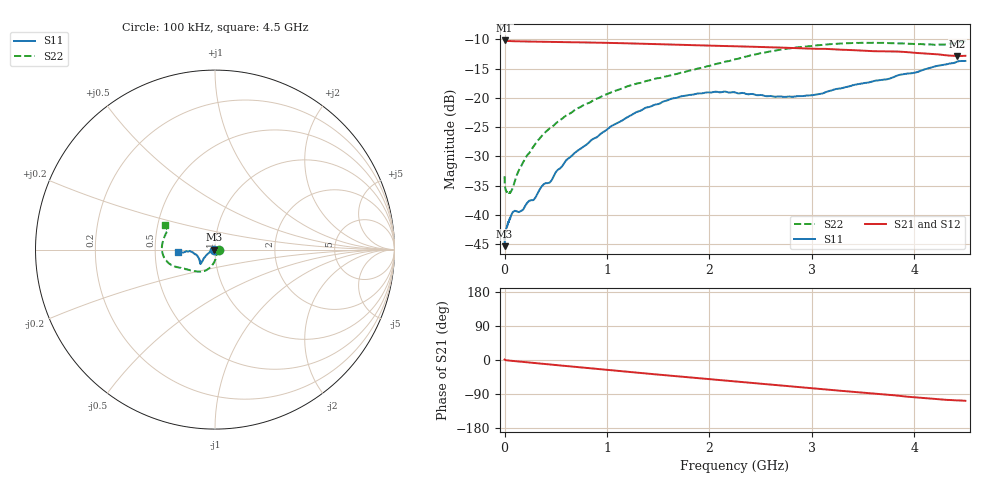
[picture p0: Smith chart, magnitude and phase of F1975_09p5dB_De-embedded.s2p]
! Integrated Device Technology
! Corporate Headquarters
! 6024 Silver Creek Valley Road
! San Jose, CA 95138  USA
! Phone:  1-408-284-8200
! Toll Free:  1-800-223-1366
! Webpage:  http://www.idt.com/
! Timing and RF Division
! 515 Groton Road, Suite 102
! Westford, MA 01886-6024
! Device:  F1975
! Description: 6-bit, 75 ohm, 0.5 dB Digital Step Attenuator
! Frequency:  5.0 MHz -  3.00 GHz
! Package:  4x4 mm QFN Plastic Package: 20 pin
! Ports:  2 RF, 11 DC
!  Pin  1  = D5 (16 dB)
!  Pin  2  = RF1  =  Port 1
!  Pin  3  = Serial Data In (DATA)
!  Pin  4  = Serial Clock (CLK)
!  Pin  5  = Serial Latch Enable (LE)
!  Pin  6  = VDD
!  Pin  7  = NC
!  Pin  8  = NC
!  Pin  9  = NC
!  Pin 10  = GND
!  Pin 11  = GND
!  Pin 12  = NC
!  Pin 13  = VMODE
!  Pin 14  = RF2  =  Port 2
!  Pin 15  = D4 (8 dB)
!  Pin 16  = D3 (4 dB)
!  Pin 17  = D2 (2 dB)
!  Pin 18  = NC
!  Pin 19  = D1 (1 dB)
!  Pin 20  = D0 (0.5 dB)
! State:  19
! Atten State:  9.5 dB
! Voltage:  +3.30 Volts
! Current:  0.563 mA
! Data:  The device was measured on a F1975 evaluation board which has
!  individual transmission lines to the RF pins.  Data was collected
!  using a calibrated network analyzer.  The evaluation board was
!  de-embedded using Automatic Fixture Removal (AFR).
!  The reference plane is the edge of the package pin.
! Misc:
!  Action Tracker AT0415
! Date Measured:  2018-02-08
! Date:  2018-03-26  MJV
! Note:
!  Integrated Device Technology supplies this data as a sample of measured
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# GHz S dB R 75
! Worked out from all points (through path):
!   291 points, 100 kHz to 4.5 GHz, reference 75 ohm
!   highest |S21| = -10.16 dB at 100 kHz (marker M1); lowest = -12.8 dB at 4.42 GHz (marker M2)
!   group delay of S21, straight-line fit = 67.8 ps
!   lowest |S11| = -45.4 dB at 100 kHz (marker M3), VSWR 1.01, Z = 74.2 - j0.00729 ohm
!   |S11| at or under -10 dB: start of sweep to end of sweep
!   |S22| runs from -36.3 to -10.2 dB; largest |S21 - S12| = 0.00018
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0.0001  -45.37 -179.5  -10.16 1.2  -10.16 1.2  -33.41 -0.4
0.0005  -44.29 -176.2  -10.18 1.1  -10.18 1.1  -34.02 -2.9
0.002  -43.51 -174.8  -10.21 0.8  -10.21 0.8  -34.88 -5.0
0.017  -42.39 -172.3  -10.25 -0.7  -10.24 -0.7  -36.01 -17.9
0.056  -40.58 -169.6  -10.28 -1.8  -10.28 -1.8  -36.21 -39.3
0.08  -39.53 -164.6  -10.29 -2.4  -10.29 -2.4  -35.43 -52.3
0.14  -39.55 -158.0  -10.32 -4.0  -10.32 -4.0  -32.37 -65.7
0.32  -36.43 -163.1  -10.37 -8.7  -10.37 -8.7  -27.35 -82.6
0.38  -34.81 -158.5  -10.39 -10.3  -10.39 -10.3  -26.22 -84.8
0.44  -34.50 -157.6  -10.41 -11.7  -10.40 -11.8  -25.21 -86.6
0.6  -30.70 -157.6  -10.45 -15.8  -10.45 -15.8  -23.01 -93.8
0.76  -28.46 -151.9  -10.50 -19.9  -10.50 -19.9  -21.35 -99.3
1.04  -24.84 -146.9  -10.59 -27.1  -10.59 -27.1  -19.04 -108.3
1.38  -21.66 -141.1  -10.74 -35.6  -10.74 -35.6  -17.12 -120.0
1.52  -20.93 -138.1  -10.78 -39.0  -10.78 -39.0  -16.58 -124.8
1.88  -19.27 -135.6  -10.99 -47.8  -10.99 -47.8  -15.00 -139.1
2.26  -19.11 -137.9  -11.16 -56.8  -11.16 -56.8  -13.35 -151.3
2.64  -19.80 -148.3  -11.35 -65.9  -11.35 -65.9  -11.93 -159.7
3.02  -19.50 -163.3  -11.57 -74.8  -11.57 -74.8  -11.06 -168.0
3.76  -16.70 -175.9  -12.02 -91.9  -12.02 -91.9  -10.62 171.9
4.42  -13.79 -174.7  -12.83 -106.5  -12.83 -106.5  -10.50 155.3
4.5  -13.67 -176.7  -12.79 -107.7  -12.79 -107.7  -10.24 154.0
